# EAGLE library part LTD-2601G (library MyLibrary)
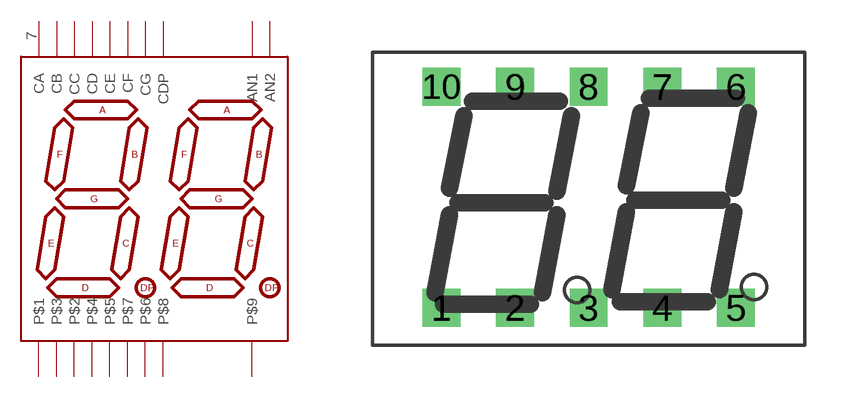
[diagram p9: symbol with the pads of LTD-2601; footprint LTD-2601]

Designator prefix -

## LTD-2601G  [LTD-2601]
1  CE
2  CD
3  CC
4  CG
5  CDP
6  AN2
7  CA
8  CB
9  AN1
10  CF

## Footprint LTD-2601 (pad centres in mm)
drill 0.8 square: 1 -5.08,-3.81; 2 -2.54,-3.81; 3 0,-3.81; 4 2.54,-3.81; 5 5.08,-3.81; 6 5.08,3.81; 7 2.54,3.81; 8 0,3.81; 9 -2.54,3.81; 10 -5.08,3.81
